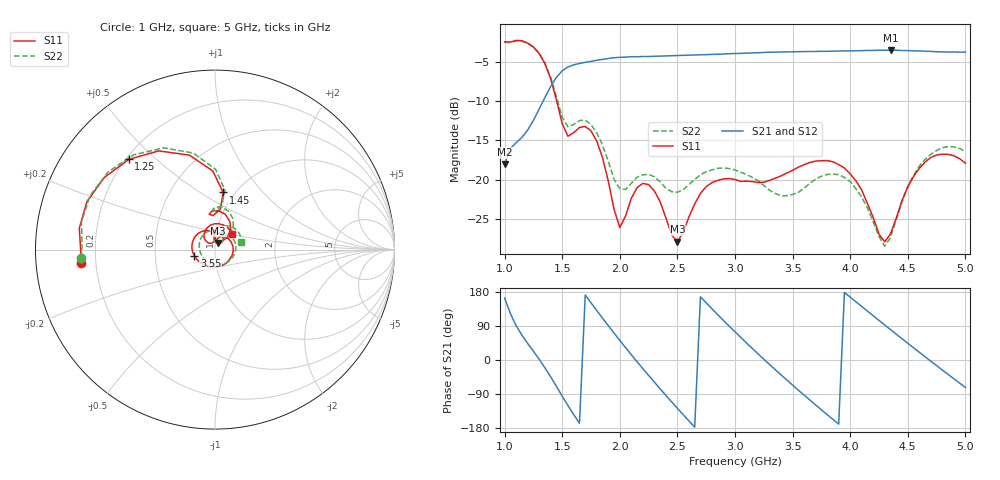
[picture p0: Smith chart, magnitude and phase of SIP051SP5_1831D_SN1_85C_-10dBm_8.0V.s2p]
# GHz  S  dB  R  50
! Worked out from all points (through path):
!   81 points, 1 GHz to 5 GHz, reference 50 ohm
!   highest |S21| = -3.55 dB at 4.35 GHz (marker M1); lowest = -18.0 dB at 1 GHz (marker M2)
!   lowest |S11| = -27.8 dB at 2.5 GHz (marker M3), VSWR 1.08, Z = 51.7 + j3.76 ohm
!   |S11| at or under -10 dB: 1.452 GHz to end of sweep
!   |S22| runs from -28.4 to -2.4 dB; largest |S21 - S12| = 0.0026
!   S11 on the Smith chart (normalised r, x): 1 GHz: 0.14, -0.05; 1.25 GHz: 0.21, +0.41; 1.45 GHz: 0.89, +0.63; 3.55 GHz: 0.79, -0.06; 5 GHz: 1.18, +0.21
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1  -2.50 -174.2  -17.99 163.6  -18.01 163.7  -2.55 -176.3
1.25  -3.16 133.7  -12.45 23.2  -12.44 23.1  -3.15 130.6
1.45  -9.86 81.9  -7.00 -69.7  -6.99 -69.7  -9.45 80.7
1.55  -14.46 93.4  -5.67 -120.3  -5.67 -120.4  -13.27 89.2
1.7  -13.23 85.1  -5.10 171.8  -5.09 171.7  -12.42 79.7
1.85  -17.19 51.2  -4.72 110.4  -4.70 110.4  -15.58 51.9
1.95  -23.71 49.1  -4.51 71.0  -4.52 71.1  -19.91 49.6
2  -26.03 72.6  -4.46 51.7  -4.44 51.7  -21.11 59.4
2.15  -20.97 88.3  -4.39 -4.6  -4.38 -4.6  -19.65 70.5
2.35  -22.76 50.3  -4.30 -75.9  -4.29 -75.9  -20.23 52.1
2.5  -27.84 63.5  -4.23 -127.4  -4.23 -127.4  -21.56 53.7
2.7  -21.72 63.8  -4.14 166.8  -4.13 166.8  -19.34 47.3
2.85  -20.05 25.2  -4.07 119.7  -4.05 119.7  -18.53 26.2
3  -19.95 -18.8  -3.98 74.5  -3.97 74.3  -18.73 -0.3
3.25  -20.29 -93.1  -3.84 2.1  -3.84 2.1  -20.70 -59.4
3.55  -18.38 -162.9  -3.74 -79.6  -3.74 -79.6  -21.57 -169.6
3.7  -17.61 165.8  -3.72 -118.6  -3.71 -118.6  -19.91 140.9
4  -19.23 108.4  -3.65 166.0  -3.64 165.9  -20.23 70.3
4.2  -24.77 88.5  -3.59 116.7  -3.58 116.8  -25.30 49.4
4.35  -26.84 129.8  -3.55 80.2  -3.58 80.2  -27.30 90.4
4.65  -17.74 109.0  -3.69 8.6  -3.69 8.5  -17.40 74.2
5  -17.88 43.3  -3.80 -72.6  -3.80 -72.7  -16.41 15.9
